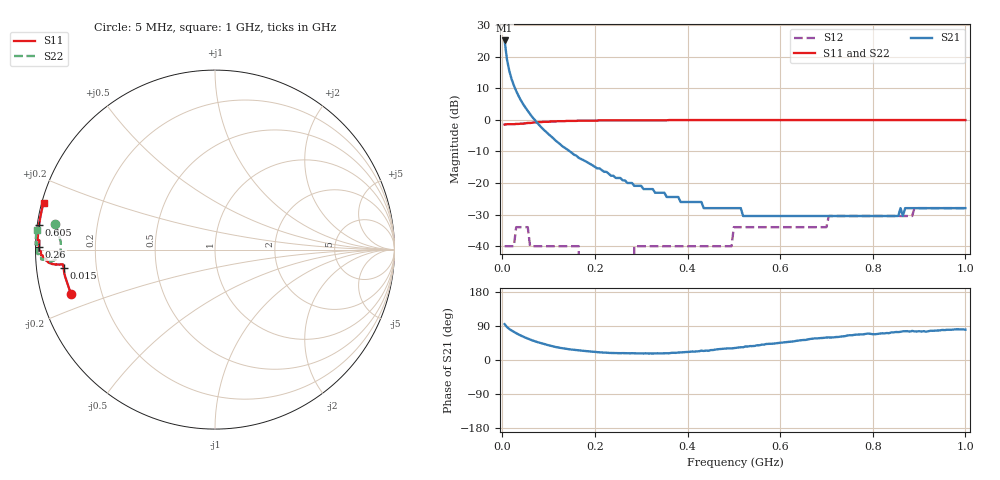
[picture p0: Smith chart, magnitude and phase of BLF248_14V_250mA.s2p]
! Filename:  BLF248_14V_250mA.s2p
! Philips part #: BLF248  !date: 22-05-2003
!Vdd=14V ; Idq=250mA
!D:\Vee measurements\measurement data\VDMOST\BLF248\14V_250mA_#1
# HZ S MA R 50
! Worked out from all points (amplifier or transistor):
!   200 points, 5 MHz to 1 GHz, reference 50 ohm
!   highest |S21| = 25.1 dB at 5 MHz (marker M1)
!   |S21| within 3 dB of that: start of sweep to 7.526 MHz
!   S11 on the Smith chart (normalised r, x): 5 MHz: 0.09, -0.15; 15 MHz: 0.08, -0.06; 260 MHz: 0.01, +0.01; 605 MHz: 0.01, +0.07; 1 GHz: 0.01, +0.13
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5000000  0.84 -162.8  17.99 94.7  0.01 3.1  0.9 171.0
1e7  0.85 -170.6  9.08 87.1  0.01 21.4  0.87 175.4
1.5e7  0.85 -173.1  6 81.9  0.01 21.7  0.86 177.2
2e7  0.85 -174.0  4.42 77.8  0.01 17.7  0.86 178.5
3e7  0.86 -174.5  2.86 70.7  0.02 7.5  0.86 -179.9
4e7  0.87 -174.5  2.04 64.5  0.02 -1.1  0.86 -178.4
5.5e7  0.89 -174.6  1.38 56.5  0.02 -11.4  0.88 -176.8
6e7  0.89 -174.7  1.23 54.0  0.01 -14.2  0.89 -176.6
9.5e7  0.93 -175.7  0.64 40.5  0.01 -27.1  0.92 -175.9
1.65e8  0.97 -178.2  0.25 25.4  0.01 -24.7  0.96 -176.7
1.7e8  0.97 -178.3  0.24 24.9  0 -22.8  0.97 -176.8
1.75e8  0.97 -178.5  0.23 24.2  0 -20.5  0.97 -176.9
2.6e8  0.98 179.1  0.11 18.2  0 58.5  0.98 -178.5
2.8e8  0.98 178.6  0.1 18.0  0 67.5  0.99 -178.8
2.85e8  0.98 178.5  0.09 17.7  0.01 69.4  0.99 -178.9
3.4e8  0.98 177.3  0.07 17.3  0.01 77.6  0.99 -179.6
4.95e8  0.99 174.2  0.04 30.5  0.01 88.6  1 178.6
5.05e8  0.99 174.0  0.04 32.1  0.02 88.5  1 178.5
6.05e8  0.99 172.1  0.03 46.1  0.02 89.2  1 177.5
6.7e8  0.99 170.9  0.03 56.2  0.02 90.4  1 176.8
8.35e8  0.99 167.8  0.03 70.8  0.03 92.6  1 175.4
1e9  0.99 164.7  0.04 80.1  0.04 91.5  1 173.8
